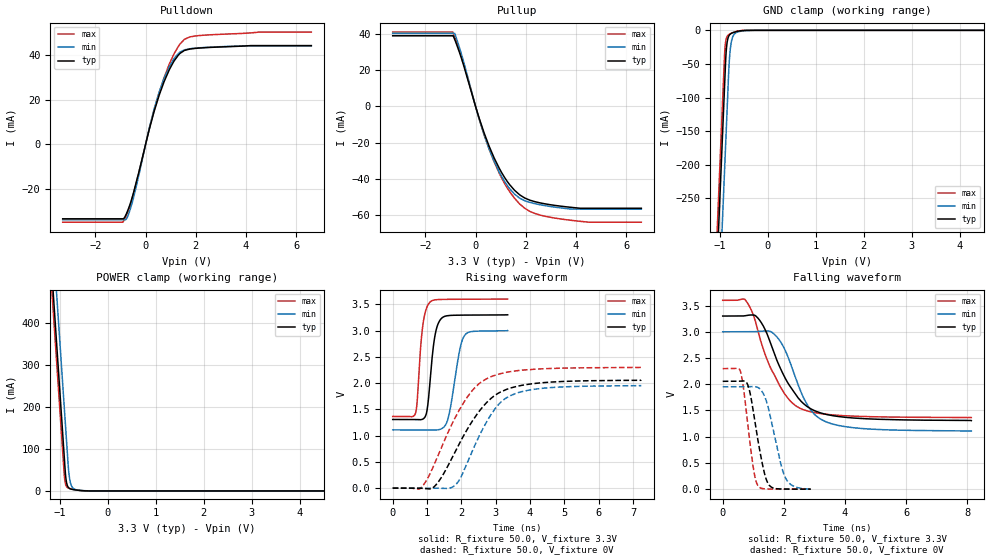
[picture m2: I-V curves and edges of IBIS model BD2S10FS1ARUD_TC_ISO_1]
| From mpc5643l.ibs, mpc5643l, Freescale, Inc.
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| *** New cell (Generated with 5.14beta1 (Sep 20 2010 13:23:23))
[Model]   BD2S10FS1ARUD_TC_ISO_1
Model_type I/O
Polarity   Non-Inverting
Enable   Active-Low
| CAP_THRESHOLD on pad pad is "CMOS" :
| Rising=10.0% of VDDE1   Falling=90.0% of VDDE1
| C_comp min and max val. don't necessarily correlate with the min and max pvt
| but are the smallest and greatest pad capacitance found.
| var   typ   min   max
C_comp   2.62627pF  2.43128pF  2.86961pF
Vinl = 1.05V | Dummy value overriden by next lines
Vinh = 2.34V | Dummy value overriden by next lines
Vmeas = 1.65V   | Reference voltage for timing measurements
Cref  = 25.0pF   | Timing specification test load capacitance value
Rref  = 1.0MOhm   | Timing specification test load resistance value
Vref  = 1.65V   | Timing specification test load voltage
[Model Spec]
| TIME_THRESHOLD on pin ipp_ind is "CORE" :
| Rising=40.0% of VDD   Falling=60.0% of VDD
Vinl 1.32350V 1.20950V 1.42250V
Vinh 1.90350V 1.72650V 2.05550V
| variable   typ   min   max
[Temperature Range] 25.0 150.0 -40.0
| variable   typ   min   max
[Voltage Range] 3.3V 3.0V 3.6V
| variable   typ   min   max
[POWER Clamp Reference] 3.3V 3.0V 3.6V
| variable   typ   min   max
[GND Clamp Reference] 0V 0V 0V
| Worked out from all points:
|   slope of the pulldown table from 0 to 0.495 V, typ, clamps not added: 24.4 ohm
|   slope of the pullup table from 0 to 0.495 V, typ, clamps not added: 24.3 ohm
|   GND clamp passes 1 mA (typ) near -0.59 V on its own axis
|   POWER clamp passes 1 mA (typ) near -0.57 V on its own axis
|   rising waveform, R_fixture 50.0, V_fixture 3.3V: 20-80 % time 187ps typ, 282ps min, 159ps max; typ from 1.31 V to 3.3 V
|   falling waveform, R_fixture 50.0, V_fixture 3.3V: 20-80 % time 1.03ns typ, 844ps min, 942ps max; typ from 3.3 V to 1.31 V
|   rising waveform, R_fixture 50.0, V_fixture 0V: 20-80 % time 1.16ns typ, 931ps min, 1.08ns max; typ from 0 V to 2.06 V
|   falling waveform, R_fixture 50.0, V_fixture 0V: 20-80 % time 367ps typ, 456ps min, 288ps max; typ from 2.06 V to 0 V
[POWER Clamp]
-3.3V     4.147A     4.265A     4.103A
-1.21V    593.6mA    712.4mA    550.2mA
-1.14V    474.6mA    593.4mA    431.2mA
-1.07V    355.6mA    474.4mA    312.2mA
-1V       236.6mA    355.4mA    193.2mA
-900mV    66.63mA    185.4mA    27.75mA
-870mV    26.01mA    134.4mA    12.15mA
-820mV    7.991mA    51.43mA    6.71mA
-790mV    5.39mA     24.66mA    5.573mA
-740mV    3.621mA    8.522mA    4.182mA
-500mV    402.7uA    702.3uA    321.1uA
6.6V      0A         0A         0A
[GND Clamp]
-3.3V     -4.159A    -4.284A    -4.112A
-1.08V    -385.3mA   -510.5mA   -337.6mA
-910mV    -96.34mA   -221.5mA   -48.6mA
-890mV    -62.34mA   -187.5mA   -23.21mA
-880mV    -45.34mA   -170.5mA   -17.17mA
-860mV    -24.34mA   -136.5mA   -10.87mA
-810mV    -7.951mA   -53.36mA   -6.135mA
-780mV    -5.416mA   -26.11mA   -4.949mA
-740mV    -3.805mA   -11.25mA   -3.696mA
-630mV    -1.487mA   -2.524mA   -1.209mA
-270mV    -802.2nA   -17.07uA   -64.06nA
6.6V      10.94nA    3.477uA    68.88pA
| variable   typ   min   max
[Pullup Reference] 3.3V 3.0V 3.6V
| variable   typ   min   max
[Pulldown Reference] 0V 0V 0V
[Pullup]
-3.3V     39.08mA    40.41mA    41.12mA
-910mV    39.08mA    40.41mA    41.12mA
-830mV    37mA       40.41mA    38.36mA
-710mV    32.57mA    35.46mA    33.89mA
-470mV    22.45mA    24.41mA    23.5mA
140mV     -6.367mA   -6.826mA   -6.792mA
740mV     -28.5mA    -30.36mA   -30.64mA
1.35V     -43.12mA   -45.36mA   -46.98mA
1.96V     -50.65mA   -52.15mA   -56.32mA
2.57V     -53.33mA   -54.36mA   -60.06mA
3.78V     -55.75mA   -56.72mA   -62.91mA
6.6V      -56.31mA   -56.78mA   -64mA
[Pulldown]
-3.3V     -33.19mA   -33.63mA   -34.7mA
-890mV    -33.19mA   -33.63mA   -34.41mA
-740mV    -30.32mA   -32.76mA   -31mA
-550mV    -24.28mA   -26.67mA   -24.8mA
-270mV    -12.48mA   -13.84mA   -12.76mA
140mV     6.42mA     6.958mA    6.662mA
340mV     14.69mA    15.77mA    15.36mA
740mV     28.08mA    29.52mA    29.87mA
1.15V     37.46mA    38.49mA    40.73mA
1.55V     41.92mA    42.17mA    46.89mA
2.57V     43.26mA    43.37mA    48.88mA
6.6V      44.08mA    43.96mA    50.1mA
[Ramp]
dV/dt_r 1.23363V/1.16238ns 1.17087V/930.57329ps 1.37887V/1.07802ns
dV/dt_f 1.19583V/1.02596ns 1.13471V/844.31713ps 1.34111V/942.33935ps
R_load = 50.0
| Removed startup time: 0s 0s 0s  .
| Removed end time: 3.348ns.
[Rising Waveform]
R_fixture   = 50.0
V_fixture   = 3.3V
V_fixture_min = 3.0V
V_fixture_max = 3.6V
0s        1.307V     1.109V     1.365V
664ps     1.307V     1.109V     1.425V
875ps     1.313V     1.109V     3.084V
994ps     1.459V     1.109V     3.442V
1.083ns   1.997V     1.108V     3.539V
1.233ns   2.909V     1.105V     3.585V
1.425ns   3.235V     1.131V     3.593V
1.626ns   3.286V     1.358V     3.595V
2.086ns   3.294V     2.899V     3.597V
3.35ns    3.3V       2.999V     3.6V
| Removed startup time: 0s 0s 0s  .
| Removed end time: 8.124ns.
[Falling Waveform]
R_fixture   = 50.0
V_fixture   = 3.3V
V_fixture_min = 3.0V
V_fixture_max = 3.6V
0s        3.3V       3V         3.6V
771ps     3.309V     3V         3.584V
996ps     3.32V      3.001V     3.329V
1.2ns     3.226V     3.008V     2.913V
1.638ns   2.66V      2.978V     2.229V
2.016ns   2.147V     2.681V     1.826V
2.559ns   1.678V     1.854V     1.533V
3.009ns   1.495V     1.421V     1.459V
3.651ns   1.396V     1.232V     1.413V
8.13ns    1.307V     1.109V     1.365V
| Removed startup time: 0s 0s 0s  .
| Removed end time: 7.239ns.
[Rising Waveform]
R_fixture   = 50.0
V_fixture   = 0V
V_fixture_min = 0V
V_fixture_max = 0V
0s        8.67nV     775.5nV    7.794nV
846ps     -3.324mV   -4.997uV   20.05mV
1.242ns   48.76mV    -934.5uV   499.1mV
1.785ns   649.3mV    37.44mV    1.297V
1.971ns   884.5mV    187.8mV    1.523V
2.268ns   1.222V     627.7mV    1.818V
2.787ns   1.661V     1.317V     2.099V
3.237ns   1.858V     1.685V     2.194V
3.879ns   1.97V      1.855V     2.252V
7.245ns   2.056V     1.951V     2.298V
| Removed startup time: 0s 0s 0s  .
| Removed end time: 2.88ns.
[Falling Waveform]
R_fixture   = 50.0
V_fixture   = 0V
V_fixture_min = 0V
V_fixture_max = 0V
0s        2.056V     1.951V     2.298V
585ps     2.061V     1.951V     2.235V
688ps     2.063V     1.951V     1.89V
853ps     1.931V     1.954V     1.069V
1.026ns   1.389V     1.956V     315.5mV
1.157ns   916mV      1.937V     62.33mV
1.475ns   117.5mV    1.587V     3.161mV
1.881ns   3.906mV    525.9mV    984.2uV
2.06ns    2.088mV    205.8mV    767.1uV
2.882ns   137.8uV    228.4uV    85.51uV
